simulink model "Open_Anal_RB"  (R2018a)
settings: Solver=ode5  StartTime=0.0  StopTime=25000  FixedStep=Tsr  RelTol=1e-3  EnableMultiTasking=on
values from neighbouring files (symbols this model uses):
  Kq1 = I22*ww^2 - 3*wo2*(I11-I33)    [start.m]    (also in run.m)
  Kq2 = 2*I22*zet*ww    [start.m]    (also in run.m)
  Kqi = 0.0005    [start.m]    (also in run.m)
  Kr1 = (0.1*I11*I33*zet^2/Hy0) - sqrt( ((0.01^zet^4*I11^2*I33^2)/Hy0^2)+(4*I11*I33*zet^2) )    [start.m]    (also in run.m)
  Kr2 = 0.05*Kr1    [start.m]    (also in run.m)
  Kr3 = 0.04*zet*(Kr2-Hy0) * sqrt(abs(Hy0/(I11*I33)))    [start.m]    (also in run.m)
  r2d = 180/pi    (= 57.2957795131)    [pl.m]    (also in pld.m; start.m; run.m; plf.m)
  Ts = 0.01    [start.m]    (also in run.m = 0.001; runf.m = 0.0005)
  Tsr = 0.01    [start.m]
  wo = 0.00113    [start.m]    (also in run.m)
undefined symbols (not defined in the file or in its folder): Arb, Brb, Crb, den, DiscIntNeverNeededParam, Drb, dsen, nsen, num, RW_Steering
libraries: simulink x3

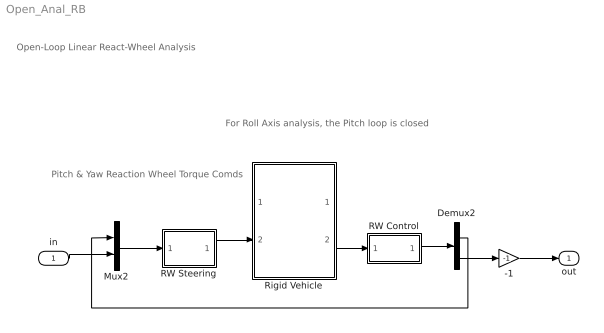
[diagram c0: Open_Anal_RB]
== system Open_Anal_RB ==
  note: Open-Loop Linear React-Wheel Analysis
  note: For Roll Axis analysis, the Pitch loop is closed
  note: Pitch & Yaw Reaction Wheel Torque Comds
  in : Inport
  -1 : Gain  Gain=-1
  Demux2 : Demux  Outputs=2
  Mux2 : Mux  Inputs=2
  RW Control : Subsystem
  RW Steering : Subsystem
  Rigid Vehicle : Subsystem
  out : Outport
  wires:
  -1/1 -> out/1
  Mux2/1 -> RW Steering/1(Trwc)
  Rigid Vehicle/2(atti) -> RW Control/1(atti)
  RW Control/1(Tc) -> Demux2/1
  RW Steering/1(Twi) -> Rigid Vehicle/2(Trw(i))
  in/1 -> Mux2/2
  Demux2/2 -> -1/1
  Demux2/1 -> Mux2/1

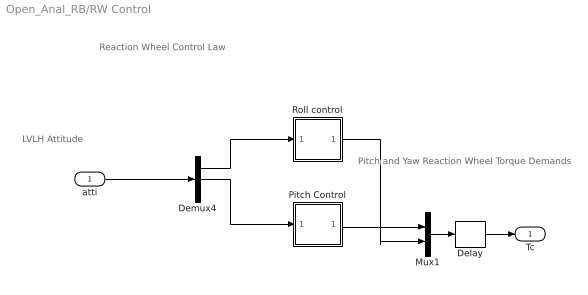
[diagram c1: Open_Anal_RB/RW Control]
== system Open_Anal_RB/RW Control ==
  note: Pitch and Yaw Reaction Wheel Torque Demands
  note: LVLH Attitude
  note: Reaction Wheel Control Law
  atti : Inport
  Delay : Delay  DelayLength=1  InputProcessing=Inherited  SampleTime=Tsr
  Demux4 : Demux  Outputs=3
  Mux1 : Mux  Inputs=2
  Pitch Control : Subsystem
  Roll control : Subsystem
  Tc : Outport
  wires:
  Demux4/1 -> Roll control/1(phi)
  Pitch Control/1(Tcy) -> Mux1/1
  Demux4/2 -> Pitch Control/1(the)
  atti/1 -> Demux4/1
  Mux1/1 -> Delay/1
  Roll control/1(Tcz) -> Mux1/2
  Delay/1 -> Tc/1

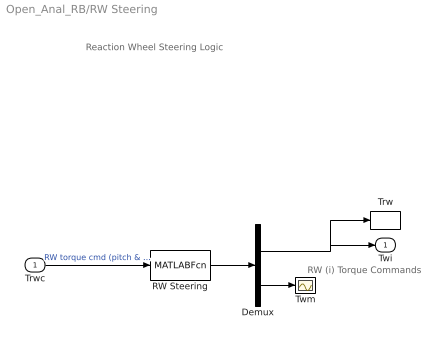
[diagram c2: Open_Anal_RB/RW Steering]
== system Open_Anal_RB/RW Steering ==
  note: RW (i) Torque Commands
  note: Reaction Wheel Steering Logic
  Trwc : Inport
  Demux : Demux  Outputs=[2, 1]
  RW Steering : MATLABFcn  MATLABFcn=RW_Steering( u(1:2) )  OutputDimensions=3
  Trw : ToWorkspace  VariableName=Trw  SampleTime=-1
  Twm : Scope
  Twi : Outport
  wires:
  Demux/2 -> Twm/1
  Demux/1 -> Twi/1, Trw/1
  RW Steering/1 -> Demux/1
  Trwc/1 -> RW Steering/1  "RW torque cmd (pitch & yaw)"

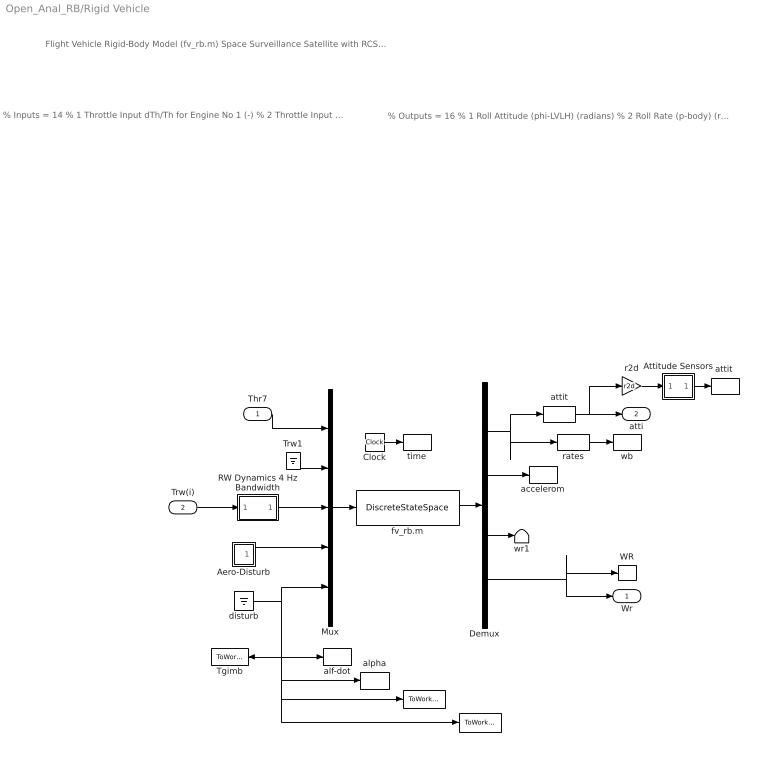
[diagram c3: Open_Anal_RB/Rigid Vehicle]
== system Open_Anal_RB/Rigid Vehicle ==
  note: % Inputs = 14 % 1 Throttle Input dTh/Th for Engine No 1 (-) % 2 Throttle Input dTh/Th for Engine No 2 (-) % 3 Throttle Input dTh/Th for Engine No 3 (-) % 4 Throttle Input dTh/Th for Engine No 4 (-) % 5 Throttle Input dTh/Th for Engine No 5 (-) % 6 Throttle Input dTh/Th for Engine No 6 (-) % 7 Throttle Input dTh/Th for Engine No 7 (-) % 8 Reaction Wheel No 1 Input Torque (ft-lb) % 9 Reaction Wheel No 2 Input Torque (ft-lb) % 10 Reaction Wheel No 3 Input Torque (ft-lb) % 11 Ext Torque Input 1 (ft-lb), dir: 1.00 0.00 0.00 % 12 Ext Torque Input 2 (ft-lb), dir: 0.00 1.00 0.00 % 13 Ext Torque Input 3 (ft-lb), dir: 0.00 0.00 1.00 % 14 Ext Torque Direct.=( 0.1970 -0.5964 -0.7782)
  note: % Outputs = 16 % 1 Roll Attitude (phi-LVLH) (radians) % 2 Roll Rate (p-body) (rad/sec) % 3 Pitch Attitude (thet-LVLH) (radians) % 4 Pitch Rate (q-body) (rad/sec) % 5 Yaw Attitude (psi-LVLH) (radians) % 6 Yaw Rate (r-body) (rad/sec) % 7 Angle of attack, alfa, (radians) % 8 Angle of sideslip, beta, (radian) % 9 Change in Altitude, delta-h, (feet) % 10 Forward Acceleration (V-dot) (ft/sec) % 11 Cross Range Velocity (Vcr) (ft/sec) % 12 Accelerom # 1, (along X), (ft/sec^2) Translat. Acceler % 13 Accelerom # 2, (along Y), (ft/sec^2) Translat. Acceler % 14 Reaction Wheel # 1 Rate (rpm) relative to vehicle % 15 Reaction Wheel # 2 Rate (rpm) relative to vehicle % 16 Reaction Wheel # 3 Rate (rpm) relative to vehicle
  note: Flight Vehicle Rigid-Body Model (fv_rb.m) Space Surveillance Satellite with RCS and Reaction Wheels (Rigid-Body)
  Thr7 : Inport
  Trw(i) : Inport  Port=2
  " " : ToWorkspace  VariableName=SA_pos  SampleTime=-1
  "   " : ToWorkspace  VariableName=SA_rate  SampleTime=-1
  Aero-Disturb : Subsystem
  Attitude Sensors : Subsystem
  Clock : Clock
  Demux : Demux  Outputs=[11, 2, 1,2]
  Mux : Mux  Inputs=[7, 1,2, 3, 1]
  RW Dynamics 4 Hz Bandwidth : Subsystem
  Tgimb : ToWorkspace  VariableName=Tgimb  SampleTime=-1
  Trw1 : Ground
  WR : ToWorkspace  VariableName=wr  SampleTime=-1
  accelerom : ToWorkspace  VariableName=accel  SampleTime=-1
  alf-dot : ToWorkspace  VariableName=alfad  SampleTime=-1
  alpha : ToWorkspace  VariableName=alfa  SampleTime=-1
  attit : Selector  InputPortWidth=11  IndexOptions=Index vector (dialog)  Indices=[1, 3, 5]  OutputSizes=1
  "attit " : ToWorkspace  VariableName=atti  SampleTime=-1
  disturb : Ground
  fv_rb.m : DiscreteStateSpace  A=Arb  B=Brb  C=Crb  D=Drb  SampleTime=Ts
  r2d : Gain  Gain=r2d
  rates : Selector  InputPortWidth=11  IndexOptions=Index vector (dialog)  Indices=[2, 4, 6]  OutputSizes=1
  time : ToWorkspace  VariableName=time  SampleTime=-1
  wb : ToWorkspace  VariableName=wb  SampleTime=-1
  wr1 : Terminator
  Wr : Outport
  atti : Outport  Port=2
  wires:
  Thr7/1 -> Mux/1
  Trw(i)/1 -> RW Dynamics 4 Hz Bandwidth/1(I)
  Demux/1 -> attit/1, rates/1
  attit/1 -> atti/1, r2d/1
  Demux/4 -> Wr/1, WR/1
  disturb/1 -> alf-dot/1, alpha/1, "   "/1, " "/1, Tgimb/1, Mux/5
  rates/1 -> wb/1
  r2d/1 -> Attitude Sensors/1(I)
  Aero-Disturb/1(Td) -> Mux/4
  Clock/1 -> time/1
  Mux/1 -> fv_rb.m/1
  fv_rb.m/1 -> Demux/1
  Demux/2 -> accelerom/1
  Trw1/1 -> Mux/2
  Demux/3 -> wr1/1
  RW Dynamics 4 Hz Bandwidth/1(O) -> Mux/3
  Attitude Sensors/1(O) -> "attit "/1

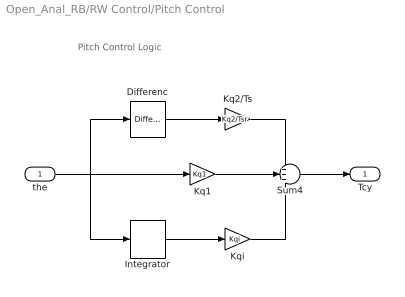
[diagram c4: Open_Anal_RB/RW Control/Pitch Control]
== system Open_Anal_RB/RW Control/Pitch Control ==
  note: Pitch Control Logic
  the : Inport
  Differenc : simulink/Discrete/Difference  ICPrevInput=0.0  InputProcessing=Inherited  OutMin=[]  OutMax=[]  OutDataType=sfix(16)  OutScaling=2^-10  DoSatur=off
  Integrator : DiscreteIntegrator  SampleTime=Tsr  ICPrevOutput=DiscIntNeverNeededParam  ICPrevScaledInput=DiscIntNeverNeededParam
  Kq1 : Gain  Gain=Kq1
  Kq2/Ts : Gain  Gain=Kq2/Tsr
  Kqi : Gain  Gain=Kqi
  Sum4 : Sum  Inputs=+++
  Tcy : Outport
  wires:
  Kq1/1 -> Sum4/2
  Sum4/1 -> Tcy/1
  Kq2/Ts/1 -> Sum4/1
  the/1 -> Kq1/1, Integrator/1, Differenc/1
  Kqi/1 -> Sum4/3
  Integrator/1 -> Kqi/1
  Differenc/1 -> Kq2/Ts/1

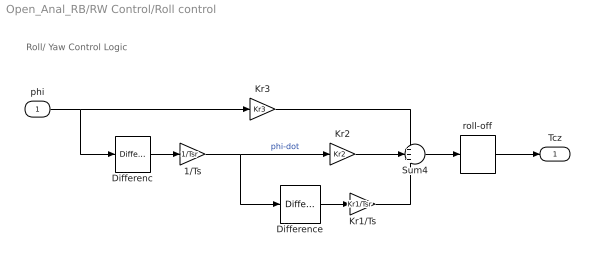
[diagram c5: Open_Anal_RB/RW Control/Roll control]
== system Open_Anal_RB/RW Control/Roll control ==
  note: Roll/ Yaw Control Logic
  phi : Inport
  1/Ts : Gain  Gain=1/Tsr
  Differenc : simulink/Discrete/Difference  ICPrevInput=0.0  InputProcessing=Inherited  OutMin=[]  OutMax=[]  OutDataType=sfix(16)  OutScaling=2^-10  DoSatur=off
  Difference : simulink/Discrete/Difference  ICPrevInput=0.0  InputProcessing=Inherited  OutMin=[]  OutMax=[]  OutDataType=sfix(16)  OutScaling=2^-10  DoSatur=off
  Kr1/Ts : Gain  Gain=Kr1/Tsr
  Kr2 : Gain  Gain=Kr2
  Kr3 : Gain  Gain=Kr3
  Sum4 : Sum  Inputs=+++
  roll-off : DiscreteTransferFcn  Numerator=[num]  Denominator=[den]  SampleTime=Tsr
  Tcz : Outport
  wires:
  roll-off/1 -> Tcz/1
  Kr3/1 -> Sum4/1
  Kr2/1 -> Sum4/2
  Kr1/Ts/1 -> Sum4/3
  phi/1 -> Kr3/1, Differenc/1
  Sum4/1 -> roll-off/1
  Difference/1 -> Kr1/Ts/1
  Differenc/1 -> 1/Ts/1
  1/Ts/1 -> Kr2/1, Difference/1  "phi-dot"

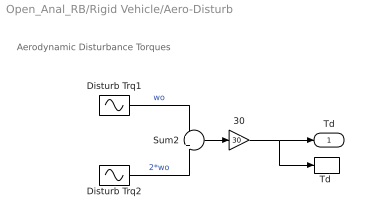
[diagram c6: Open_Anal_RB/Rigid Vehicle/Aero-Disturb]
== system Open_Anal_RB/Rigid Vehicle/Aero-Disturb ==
  note: Aerodynamic Disturbance Torques
  30 : Gain  Gain=30
  Disturb Trq1 : Sin  Amplitude="[0.0,   1,   0.2]*0.0001"  Bias="[0.0,  0.5,  0.15]*0.0001"  Frequency=[wo, wo, wo]  SampleTime=0
  Disturb Trq2 : Sin  Amplitude=[0, 1.2, 1]*0.0001  Bias=[0 0 0]  Frequency=[wo, wo, wo]*2  SampleTime=0
  Sum2 : Sum  Inputs=+|+
  "Td " : ToWorkspace  VariableName=Td  SampleTime=-1
  Td : Outport
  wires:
  30/1 -> "Td "/1, Td/1
  Disturb Trq2/1 -> Sum2/2  "2*wo"
  Sum2/1 -> 30/1
  Disturb Trq1/1 -> Sum2/1  "wo"

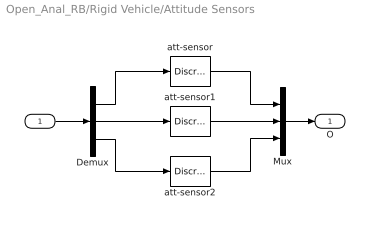
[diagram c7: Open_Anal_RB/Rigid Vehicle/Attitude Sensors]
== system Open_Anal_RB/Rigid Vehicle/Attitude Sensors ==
  I : Inport
  Demux : Demux  Outputs=3
  Mux : Mux  Inputs=3
  att-sensor : DiscreteTransferFcn  Numerator=[nsen]  Denominator=[dsen]  SampleTime=Ts
  att-sensor1 : DiscreteTransferFcn  Numerator=[nsen]  Denominator=[dsen]  SampleTime=Ts
  att-sensor2 : DiscreteTransferFcn  Numerator=[nsen]  Denominator=[dsen]  SampleTime=Ts
  O : Outport
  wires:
  I/1 -> Demux/1
  Mux/1 -> O/1
  att-sensor/1 -> Mux/1
  Demux/1 -> att-sensor/1
  Demux/3 -> att-sensor2/1
  att-sensor2/1 -> Mux/3
  Demux/2 -> att-sensor1/1
  att-sensor1/1 -> Mux/2

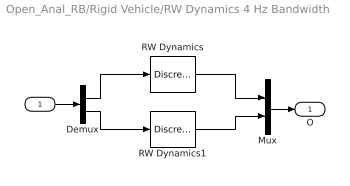
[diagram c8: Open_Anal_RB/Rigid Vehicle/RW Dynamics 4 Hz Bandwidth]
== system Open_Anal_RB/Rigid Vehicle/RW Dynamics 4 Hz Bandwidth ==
  I : Inport
  Demux : Demux  Outputs=2
  Mux : Mux  Inputs=2
  RW Dynamics : DiscreteTransferFcn  Numerator="[0  0.221199217]"  Denominator=[1 -0.778800783]  SampleTime=Ts
  RW Dynamics1 : DiscreteTransferFcn  Numerator="[0  0.221199217]"  Denominator=[1 -0.778800783]  SampleTime=Ts
  O : Outport
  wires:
  Demux/2 -> RW Dynamics1/1
  Demux/1 -> RW Dynamics/1
  I/1 -> Demux/1
  Mux/1 -> O/1
  RW Dynamics/1 -> Mux/1
  RW Dynamics1/1 -> Mux/2
